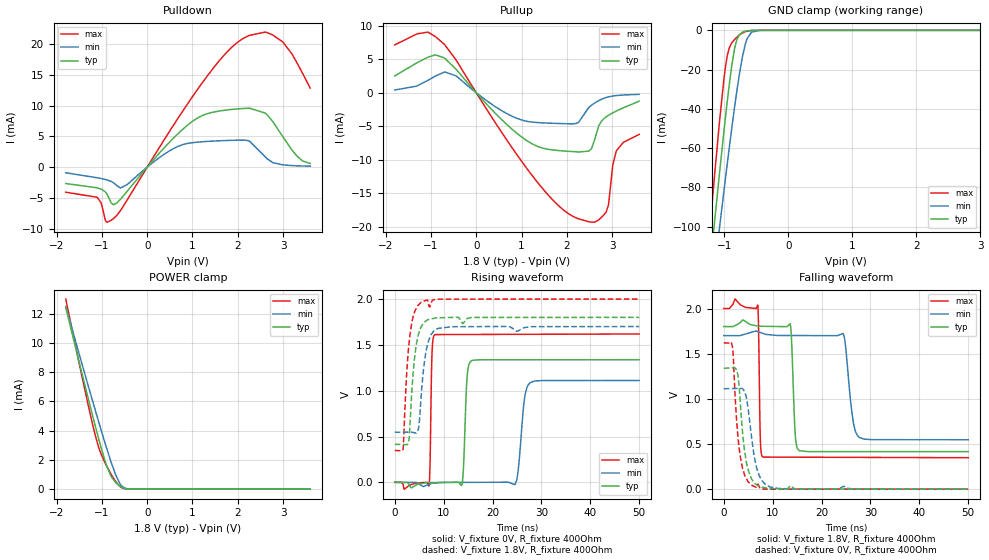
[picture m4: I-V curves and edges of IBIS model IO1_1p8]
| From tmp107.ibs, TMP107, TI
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|   Model
[Model]   IO1_1p8
Model_type   I/O
Polarity   Non-Inverting
Enable   Active-Low
Vinl = 0.54
Vinh = 1.26
Vmeas = 0.9
Vref = 0
Cref = 1pF
Rref = 100000
|   typ   min   max
C_comp   1.027pF   0.994pF   1.056pF
[Voltage Range]   1.8   1.7   2
[Temperature Range]   25   125   -55
[Pullup Reference]   1.8   1.7   2
[Pulldown Reference]   0   -0   0
[Power Clamp Reference]   1.8   1.7   2
[GND Clamp Reference]   0   0   0
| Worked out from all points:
|   slope of the pulldown table from 0 to 0.27 V, typ, clamps not added: 118 ohm
|   slope of the pullup table from 0 to 0.27 V, typ, clamps not added: 135 ohm
|   GND clamp passes 1 mA (typ) near -0.72 V on its own axis
|   POWER clamp passes 1 mA (typ) near -0.82 V on its own axis
|   falling waveform, V_fixture 1.8V, R_fixture 400Ohm: 20-80 % time 564ps typ, 1.28ns min, 268ps max; typ from 1.8 V to 0.415 V
|   rising waveform, V_fixture 0V, R_fixture 400Ohm: 20-80 % time 554ps typ, 1.06ns min, 295ps max; typ from 0 V to 1.34 V
|   rising waveform, V_fixture 1.8V, R_fixture 400Ohm: 20-80 % time 1.3ns typ, 1.36ns min, 1.29ns max; typ from 0.415 V to 1.8 V
|   falling waveform, V_fixture 0V, R_fixture 400Ohm: 20-80 % time 1.51ns typ, 1.8ns min, 1.41ns max; typ from 1.34 V to 0 V
[Pulldown]
|   Voltage   I(typ)   I(min)   I(max)
-1.8V     -2.667mA   -915.9uA   -4.078mA
-1.109V   -3.363mA   -1.727mA   -4.903mA
-909mV    -4.178mA   -2.037mA   -8.842mA
-747mV    -6.123mA   -2.523mA   -8.379mA
-590.4mV  -5.226mA   -3.393mA   -7.075mA
462.6mV   3.837mA    2.519mA    5.47mA
997.2mV   7.442mA    3.982mA    11.44mA
1.748V    9.298mA    4.335mA    18.63mA
2.255V    9.593mA    4.243mA    21.44mA
2.639V    8.605mA    1.43mA     21.93mA
2.995V    4.955mA    375.9uA    20.37mA
3.6V      590.1uA    156.3uA    12.89mA
[GND Clamp]
|   Voltage   I(typ)   I(min)   I(max)
-1.8V     -318.1mA   -308.4mA   -326.4mA
-1.222V   -120.3mA   -141.4mA   -99.5mA
-1.152V   -97.2mA    -121.7mA   -73.42mA
-1.076V   -72.88mA   -100.7mA   -46.65mA
-1.006V   -51.16mA   -81.64mA   -24.65mA
-952.2mV  -35.44mA   -67.3mA    -12.54mA
-838.8mV  -9.184mA   -38.75mA   -4.601mA
-801mV    -4.515mA   -30.01mA   -3.39mA
-720mV    -973.8uA   -13.81mA   -1.402mA
-644.4mV  -251uA     -4.197mA   -397.9uA
-444.6mV  -2.811uA   -30.12uA   -2.049uA
3.6V      0A         0A         0A
[Pullup]
|   Voltage   I(typ)   I(min)   I(max)
-1.8V     2.51mA     410.1uA    7.13mA
-1.071V   5.28mA     1.835mA    9.033mA
-714.6mV  5.211mA    3.045mA    7.269mA
1.067V    -6.904mA   -4.18mA    -10.82mA
1.748V    -8.566mA   -4.564mA   -16.37mA
2.266V    -8.823mA   -4.369mA   -18.79mA
2.542V    -8.373mA   -1.877mA   -19.28mA
2.86V     -3.637mA   -729.4uA   -17.87mA
2.92V     -3.365mA   -615.9uA   -16.76mA
3.017V    -2.994mA   -489uA     -10.75mA
3.092V    -2.738mA   -423.4uA   -8.713mA
3.6V      -1.259mA   -243.5uA   -6.207mA
[POWER Clamp]
|   Voltage   I(typ)   I(min)   I(max)
-1.8V     12.41mA    12.49mA    12.99mA
-1.298V   6.128mA    6.997mA    5.65mA
-1.163V   4.498mA    5.551mA    3.857mA
-1.071V   3.426mA    4.583mA    2.841mA
-1.022V   2.879mA    4.078mA    2.424mA
-919.8mV  1.814mA    3.032mA    1.724mA
-811.8mV  961.9uA    1.983mA    1.093mA
-693mV    440.4uA    956.6uA    513.3uA
-579.6mV  145.7uA    277.2uA    137.6uA
-444.6mV  12.78uA    26.71uA    6.027uA
-342mV    884.5nA    3.012uA    188.2nA
3.6V      0A         0A         0A
[Ramp]
R_load = 400
|   typ   min   max
dV/dt_r   0.802689/5.52967e-10   0.666748/1.05584e-09   0.971371/2.94402e-10
dV/dt_f   0.83113/5.6251e-10   0.692092/1.27598e-09   0.991465/2.67915e-10
[Falling Waveform]
V_fixture = 1.8V
V_fixture_min = 1.7V
V_fixture_max = 2V
R_fixture = 400Ohm
C_fixture = 0F
|   Time   V(typ)   V(min)   V(max)
0s        1.8V       1.7V       2V
6.942ns   1.805V     1.744V     2.038V
7.477ns   1.804V     1.734V     553.3mV
7.982ns   1.803V     1.724V     354.7mV
13.61ns   1.825V     1.701V     353.7mV
14.62ns   600mV      1.701V     353.5mV
15.43ns   425.8mV    1.701V     353.4mV
24.44ns   415.2mV    1.72V      351.9mV
27.81ns   415.2mV    570.3mV    351.3mV
50ns      414.8mV    546.5mV    347.6mV
[Rising Waveform]
V_fixture = 0V
V_fixture_min = 0V
V_fixture_max = 0V
R_fixture = 400Ohm
C_fixture = 0F
|   Time   V(typ)   V(min)   V(max)
0s        145.9nV    244.6nV    103.4nV
7.02ns    -2.834mV   -21.74mV   -36mV
7.62ns    -2.411mV   -11.04mV   1.408V
8.211ns   -1.994mV   -8.587mV   1.612V
13.73ns   -24.87mV   -594.7uV   1.613V
14.8ns    1.149V     -410.8uV   1.613V
15.75ns   1.329V     -245.8uV   1.614V
24.61ns   1.337V     -22.18mV   1.615V
27.81ns   1.337V     1.09V      1.615V
50ns      1.338V     1.111V     1.619V
[Rising Waveform]
V_fixture = 1.8V
V_fixture_min = 1.7V
V_fixture_max = 2V
R_fixture = 400Ohm
C_fixture = 0F
|   Time   V(typ)   V(min)   V(max)
0s        414.8mV    546.5mV    347.6mV
1.695ns   412.2mV    546.6mV    363.1mV
2.305ns   411.2mV    546.7mV    1.061V
2.806ns   426.8mV    546.7mV    1.455V
3.999ns   1.335V     540.8mV    1.852V
4.895ns   1.62V      598.2mV    1.939V
5.45ns    1.701V     976mV      1.968V
6.887ns   1.776V     1.542V     1.953V
8.898ns   1.796V     1.68V      2V
50ns      1.8V       1.7V       2V
[Falling Waveform]
|Gnd
V_fixture = 0V
V_fixture_min = 0V
V_fixture_max = 0V
R_fixture = 400Ohm
C_fixture = 0F
|   Time   V(typ)   V(min)   V(max)
0s        1.338V     1.111V     1.619V
1.78ns    1.343V     1.113V     1.571V
2.742ns   1.294V     1.115V     680.2mV
3.339ns   986.3mV    1.115V     371.1mV
4.219ns   436mV      1.083V     163.4mV
4.895ns   235.3mV    925.6mV    88.81mV
5.836ns   100.5mV    511mV      38.89mV
7.271ns   29.36mV    146.4mV    24.95mV
9.388ns   6.504mV    25.34mV    270.8uV
50ns      373.9nV    606.4nV    210.6nV
